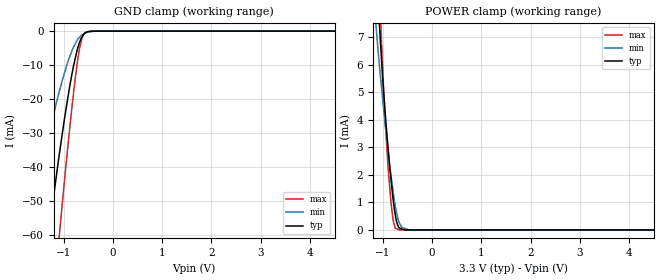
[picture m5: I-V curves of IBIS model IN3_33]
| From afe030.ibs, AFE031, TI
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|   IN3 3.3V Model
[Model]  IN3_33
Model_type Input
Vinl = 0.99
Vinh = 2.31
|   typ   min   max
|   (nom PVT)   (Fast PVT)   (slow PVT)
C_comp   2.7615410e-12  2.1504140e-12  3.3502790e-12
| Where   nom PVT is  Nominal Process, 3.3V, 52C
|   Fast PVT is Strong Process, 3.6V, -40C
|   Slow PVT is Weak Process, 3.0V, 150C
[Voltage Range]   3.3   3   3.6
[Temperature Range]   52   150   -40
[Power Clamp Reference]   3.3   3   3.6
[GND Clamp Reference]   0   0   0
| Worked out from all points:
|   GND clamp passes 1 mA (typ) near -0.60 V on its own axis
|   POWER clamp passes 1 mA (typ) near -0.78 V on its own axis
[GND Clamp]
|   Voltage   I(typ)   I(min)   I(max)
-3.3V     -329.1mA   -209.8mA   -432.2mA
-1.692V   -108mA     -59.25mA   -160mA
-1.34V    -64.25mA   -33.36mA   -101mA
-1.274V   -56.72mA   -28.95mA   -90.23mA
-1.099V   -37.41mA   -18.45mA   -61.98mA
-1.065V   -33.93mA   -16.54mA   -56.49mA
-878.9mV  -16.42mA   -7.609mA   -28.91mA
-813.5mV  -11.29mA   -5.133mA   -19.99mA
-712.8mV  -4.93mA    -2.399mA   -8.233mA
-632.3mV  -1.786mA   -1.159mA   -2.35mA
-556.4mV  -431.9uA   -525.4uA   -392.4uA
6.6V      0A         0A         0A
[POWER Clamp]
|   Voltage   I(typ)   I(min)   I(max)
-3.3V     97.53mA    76.89mA    125.2mA
-1.135V   9.633mA    7.32mA     11.73mA
-1.063V   7.267mA    5.838mA    8.425mA
-1.055V   7.016mA    5.684mA    8.072mA
-1.028V   6.214mA    5.186mA    6.855mA
-969.9mV  4.677mA    4.142mA    4.573mA
-885.7mV  2.805mA    2.76mA     2.084mA
-817mV    1.53mA     1.74mA     709.6uA
-743.4mV  495.9uA    821.4uA    60.57uA
-658.7mV  68.03uA    223uA      1.48uA
-465.3mV  1.886uA    2.393uA    1.441uA
6.6V      0A         0A         0A
